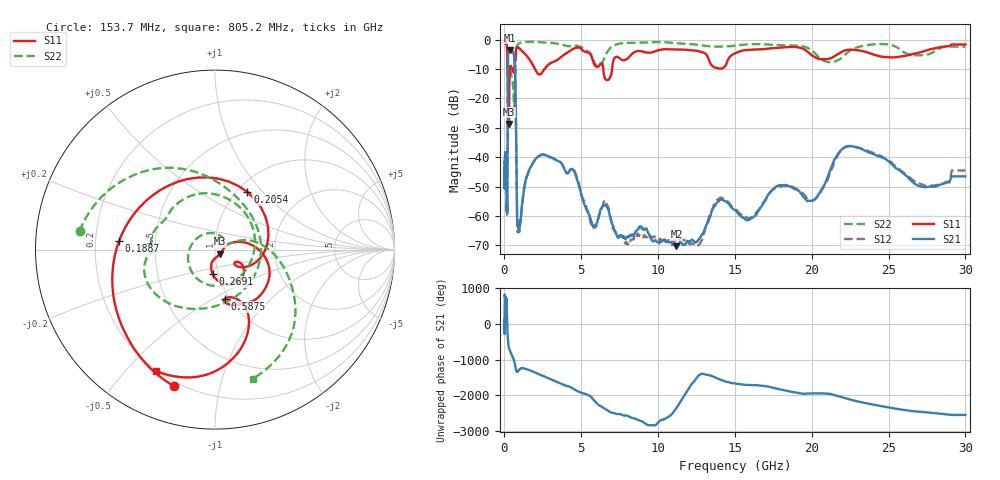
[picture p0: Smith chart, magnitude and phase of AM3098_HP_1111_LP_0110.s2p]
! Date/Time: Thu, Feb 28, 2019 8:47 AM
! Network Analyzer: Agilent Technologies E8364B Rev: A.07.50.67
! Sweep from 0.010 to 30.000 GHz, 1601 Points, Sweep Type: LOG
! Power Supply: 5.022 V, 0.002 A
# Hz S DB R 50
!freq MagS11 AngS11 MagS21 AngS21 MagS12 AngS12 MagS22 AngS22
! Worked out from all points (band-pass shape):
!   1601 points, 10 MHz to 30 GHz, reference 50 ohm
!   highest |S21| = -3.43 dB at 340.5 MHz (marker M1); lowest = -70.3 dB at 11.19 GHz (marker M2)
!   |S21| within 3 dB of the highest: 228.1 MHz to 645.6 MHz (417.5 MHz wide, 95.6 % of centre)
!   lowest |S11| = -28.7 dB at 290.1 MHz (marker M3), VSWR 1.08, Z = 52.9 - j2.46 ohm
!   |S11| at or under -10 dB: 210 MHz to 353.9 MHz (143.9 MHz wide, 51 % of centre); 1.994 GHz to 2.601 GHz (606.4 MHz wide, 26.4 % of centre); 6.433 GHz to 7.005 GHz (571.6 MHz wide, 8.51 % of centre)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
!   |S22| runs from -23.4 to -0.5 dB; largest |S21 - S12| = 0.01
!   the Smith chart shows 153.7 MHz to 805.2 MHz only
!   S11 on the Smith chart (normalised r, x): 153.7 MHz: 0.18, -0.73; 188.7 MHz: 0.30, +0.04; 205.4 MHz: 1.12, +0.83; 269.1 MHz: 0.94, -0.26; 587.5 MHz: 0.95, -0.57; 805.2 MHz: 0.20, -0.61
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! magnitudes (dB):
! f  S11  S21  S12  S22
! 10 MHz  -0.3  -43.4  -41.2  -0.5
! 38.04 MHz  -0.2  -40.9  -41.1  -0.6
! 96 MHz  -0.8  -39.8  -39.3  -1.3
! 144.7 MHz  -1.6  -54.5  -56.7  -2.0
! 153.7 MHz  -2.0  -58.1  -56.7  -2.4
! 188.7 MHz  -5.4  -54.3  -52.2  -9.3
! 205.4 MHz  -8.7  -23.4  -23.5  -9.6
! 269.1 MHz  -17.3  -3.9  -3.9  -9.0
! 290.1 MHz  -28.7  -3.6  -3.6  -9.6
! 340.5 MHz  -11.1  -3.4  -3.4  -9.6
! 550.5 MHz  -10.5  -4.2  -4.2  -15.4
! 587.5 MHz  -11.1  -4.6  -4.6  -19.0
! 703.4 MHz  -5.7  -12.7  -12.7  -11.4
! 805.2 MHz  -2.5  -54.6  -55.0  -2.5
! 964.1 MHz  -2.9  -65.5  -63.4  -1.2
! 2.084 GHz  -10.9  -40.3  -40.3  -0.8
! 4.458 GHz  -3.1  -44.2  -43.9  -2.0
! 7.926 GHz  -6.7  -67.5  -68.8  -1.1
! 11.19 GHz  -3.3  -70.3  -68.7  -1.1
! 20.1 GHz  -5.6  -54.6  -54.7  -4.1
! 22.56 GHz  -3.4  -36.2  -36.2  -3.5
! 30 GHz  -1.6  -46.5  -44.5  -2.3
